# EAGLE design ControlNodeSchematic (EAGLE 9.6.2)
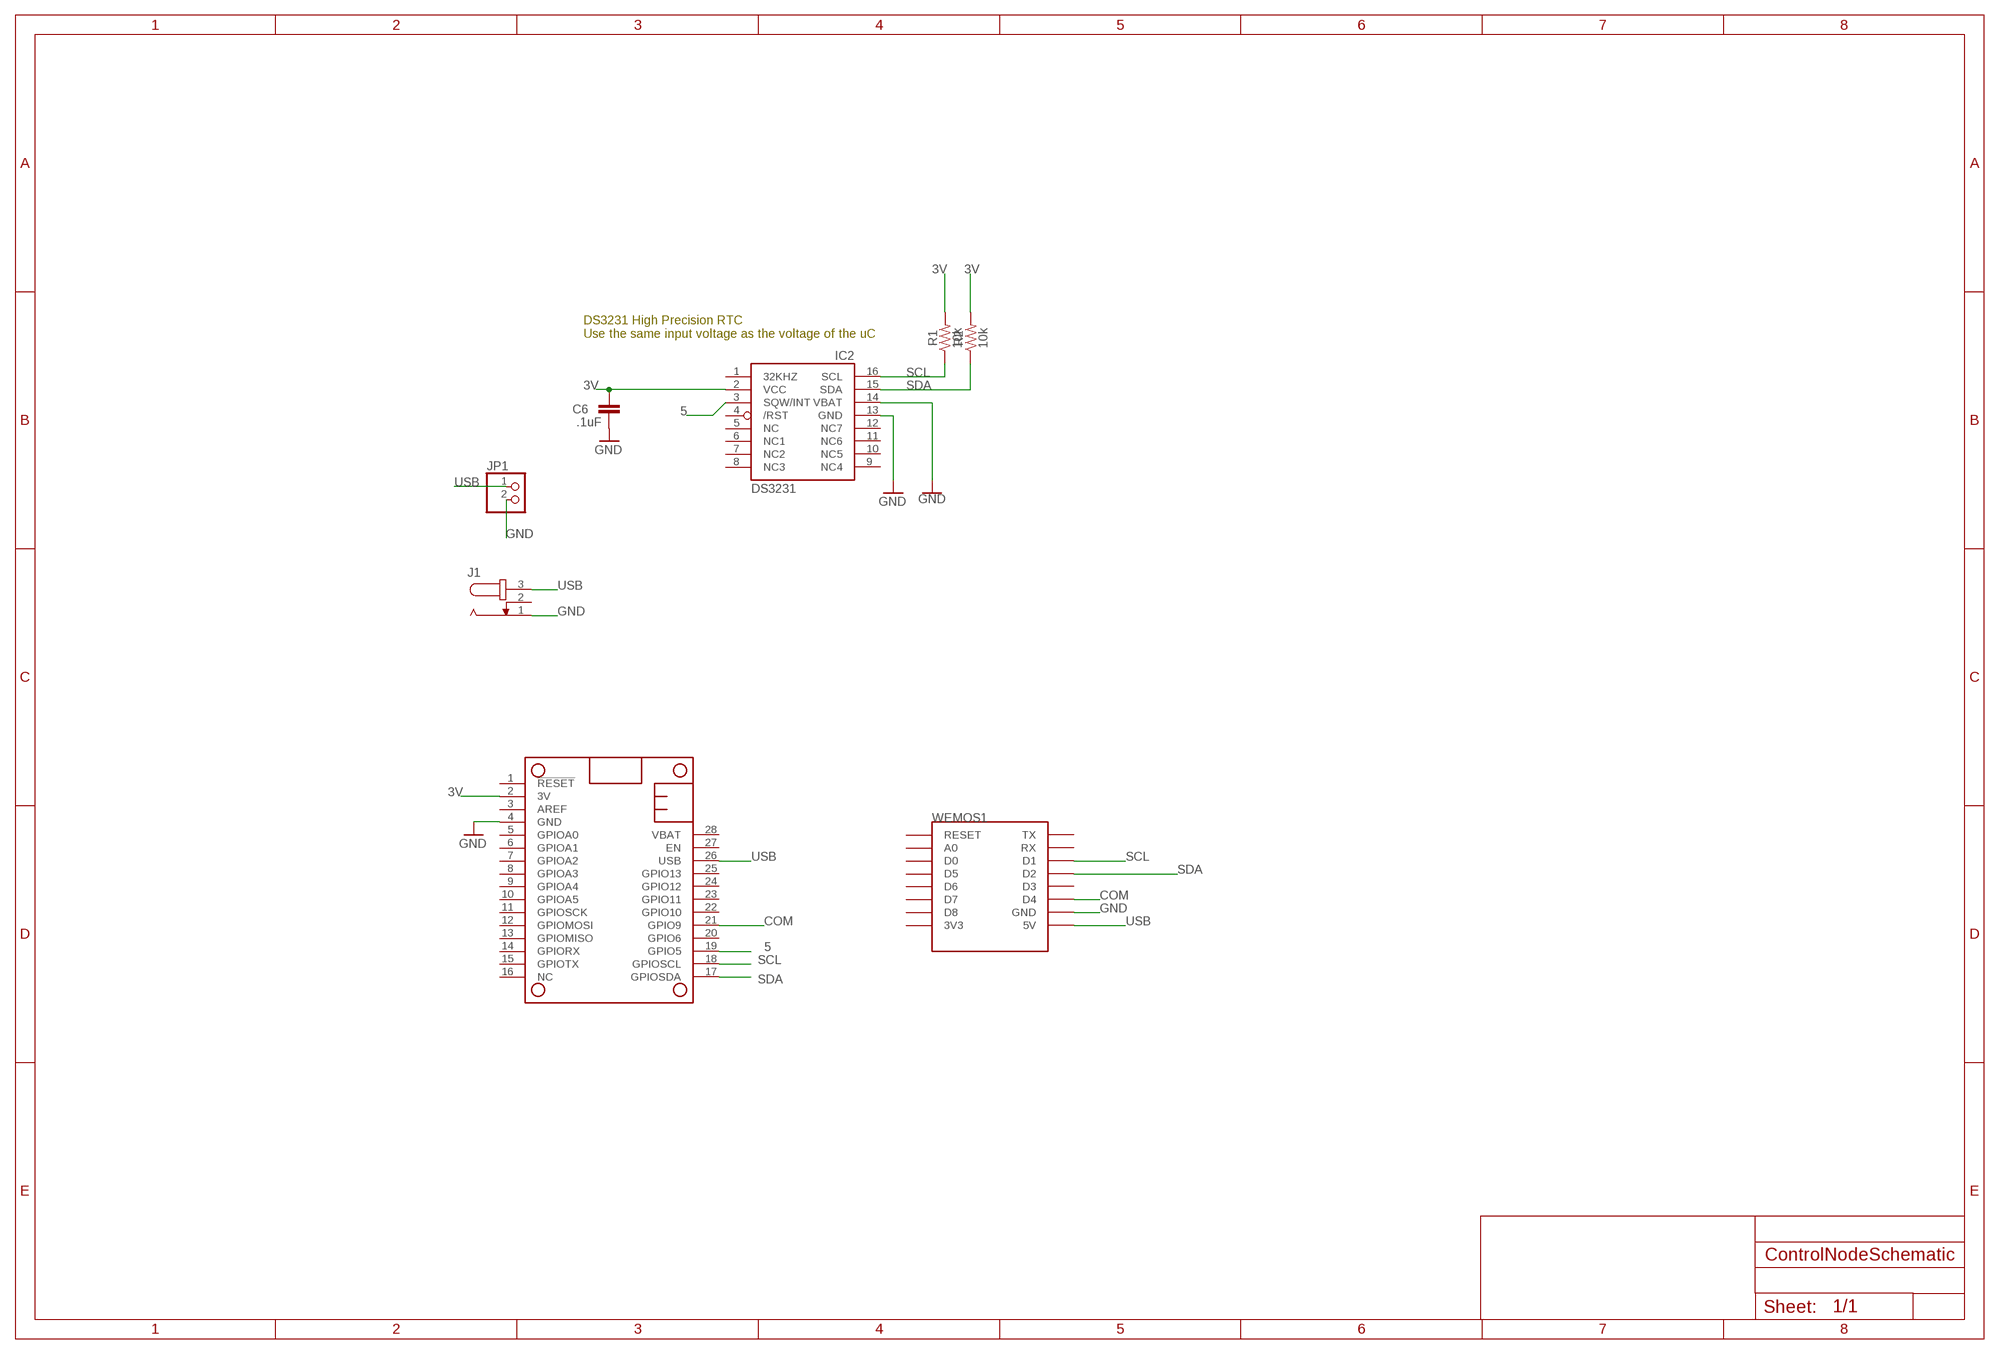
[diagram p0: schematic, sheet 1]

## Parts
C6  .1uF  CC1206  [C1206]
IC2  DS3231/SO  [SO16W]
J1  JACK-PLUG1  [SPC4078]
JP1  PINHD-1X2  [1X02]
MS1  FEATHERWING_NODIM  [FEATHERWING_DIM]
R1  10k  0.27OHM-0603-1/10W-1%  [0603]
R2  10k  0.27OHM-0603-1/10W-1%  [0603]
WEMOS1  WEMOS-D1-MINI  [WEMOS-D1-MINI]

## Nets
3V: C6.1 IC2.2(VCC) MS1.2(3V) R1.2 R2.2
5: IC2.3(SQW/INT) MS1.19(GPIO5)
COM: MS1.21(GPIO9) WEMOS1.D4
GND: C6.2 IC2.13(GND) IC2.14(VBAT) J1.1 JP1.2 MS1.4(GND) WEMOS1.GND
SCL: IC2.16(SCL) MS1.18(GPIOSCL) R1.1 WEMOS1.D1
SDA: IC2.15(SDA) MS1.17(GPIOSDA) R2.1 WEMOS1.D2
USB: J1.3 JP1.1 MS1.26(USB) WEMOS1.5V
Unconnected: IC2.1(32KHZ) IC2.4(/RST) IC2.5(NC) IC2.6(NC1) IC2.7(NC2) IC2.8(NC3) IC2.9(NC4) IC2.10(NC5) IC2.11(NC6) IC2.12(NC7) J1.2 MS1.1(!RESET) MS1.3(AREF) MS1.5(GPIOA0) MS1.6(GPIOA1) MS1.7(GPIOA2) MS1.8(GPIOA3) MS1.9(GPIOA4) MS1.10(GPIOA5) MS1.11(GPIOSCK) MS1.12(GPIOMOSI) MS1.13(GPIOMISO) MS1.14(GPIORX) MS1.15(GPIOTX) MS1.16(NC) MS1.20(GPIO6) MS1.22(GPIO10) MS1.23(GPIO11) MS1.24(GPIO12) MS1.25(GPIO13) MS1.27(EN) MS1.28(VBAT) WEMOS1.3V3 WEMOS1.A0 WEMOS1.D0 WEMOS1.D3 WEMOS1.D5 WEMOS1.D6 WEMOS1.D7 WEMOS1.D8 WEMOS1.RESET WEMOS1.RX WEMOS1.TX

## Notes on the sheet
- DS3231 High Precision RTC
  Use the same input voltage as the voltage of the uC

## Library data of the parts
C6 = eagle-ltspice:C: CAPACITOR, European symbol; SPICEMODEL: NONE; SPICEPREFIX: C
IC2 = adafruit:DS3231
J1 = con-jack:JACK-PLUG: DC POWER JACK Power Jack, DC, Right Angle, Through Hole, Rated 5A at 16VDC, PC Terminals Distributor: Farnell (www.Farnell.de) Drawing: 84N1161.pdf / 84N1162.pdf Manufacturer: SPC Technology (www.spctechnology.com) Type: SPC4077 / SPC 4078; OC_FARNELL: unknown; OC_NEWARK: unknown
JP1 = pinhead:PINHD-1X2: PIN HEADER
MS1 = adafruit:FEATHERWING
R1 R2 = SparkFun-Resistors:0.27OHM: 0.27Ω resistor; PROD_ID: RES-08787; VALUE: 0.27
WEMOS1 = esp8266modules:WEMOS-D1-MINI: WeMos.cc D1 mini ESP8266 module

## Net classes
0 default: width 0.203 mm, drill 0.203 mm, clearance 0.178 mm

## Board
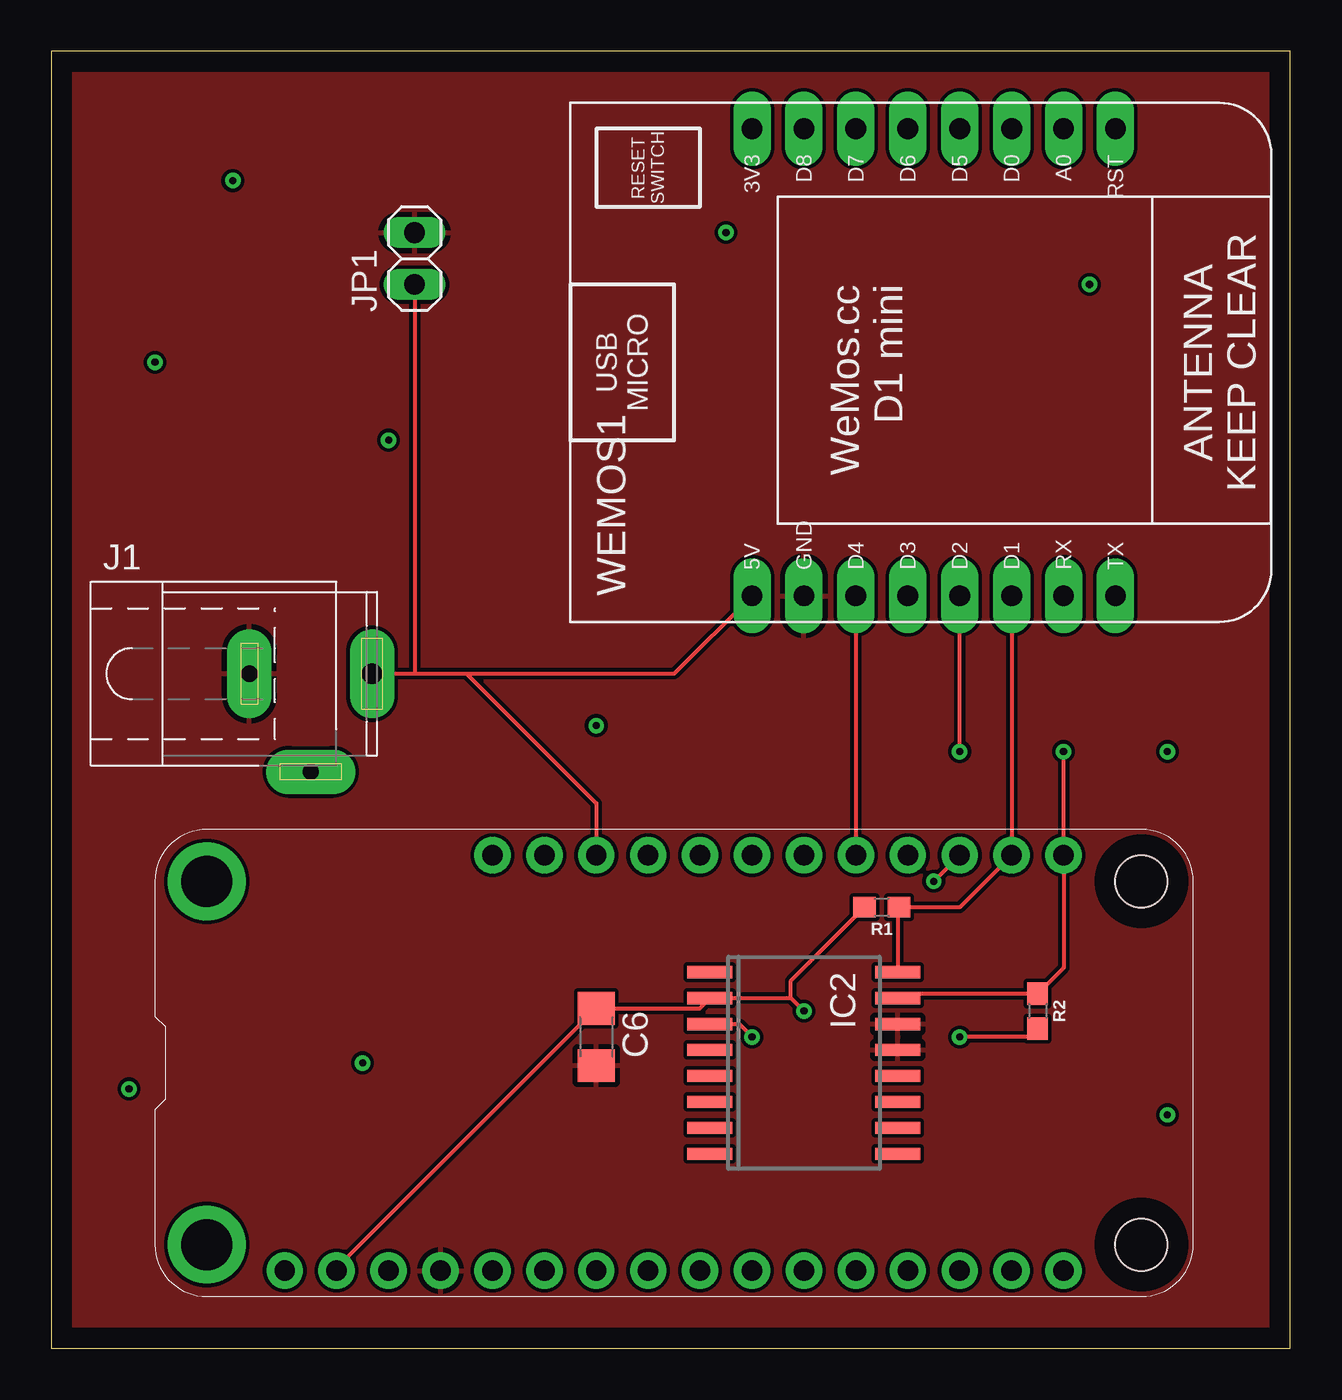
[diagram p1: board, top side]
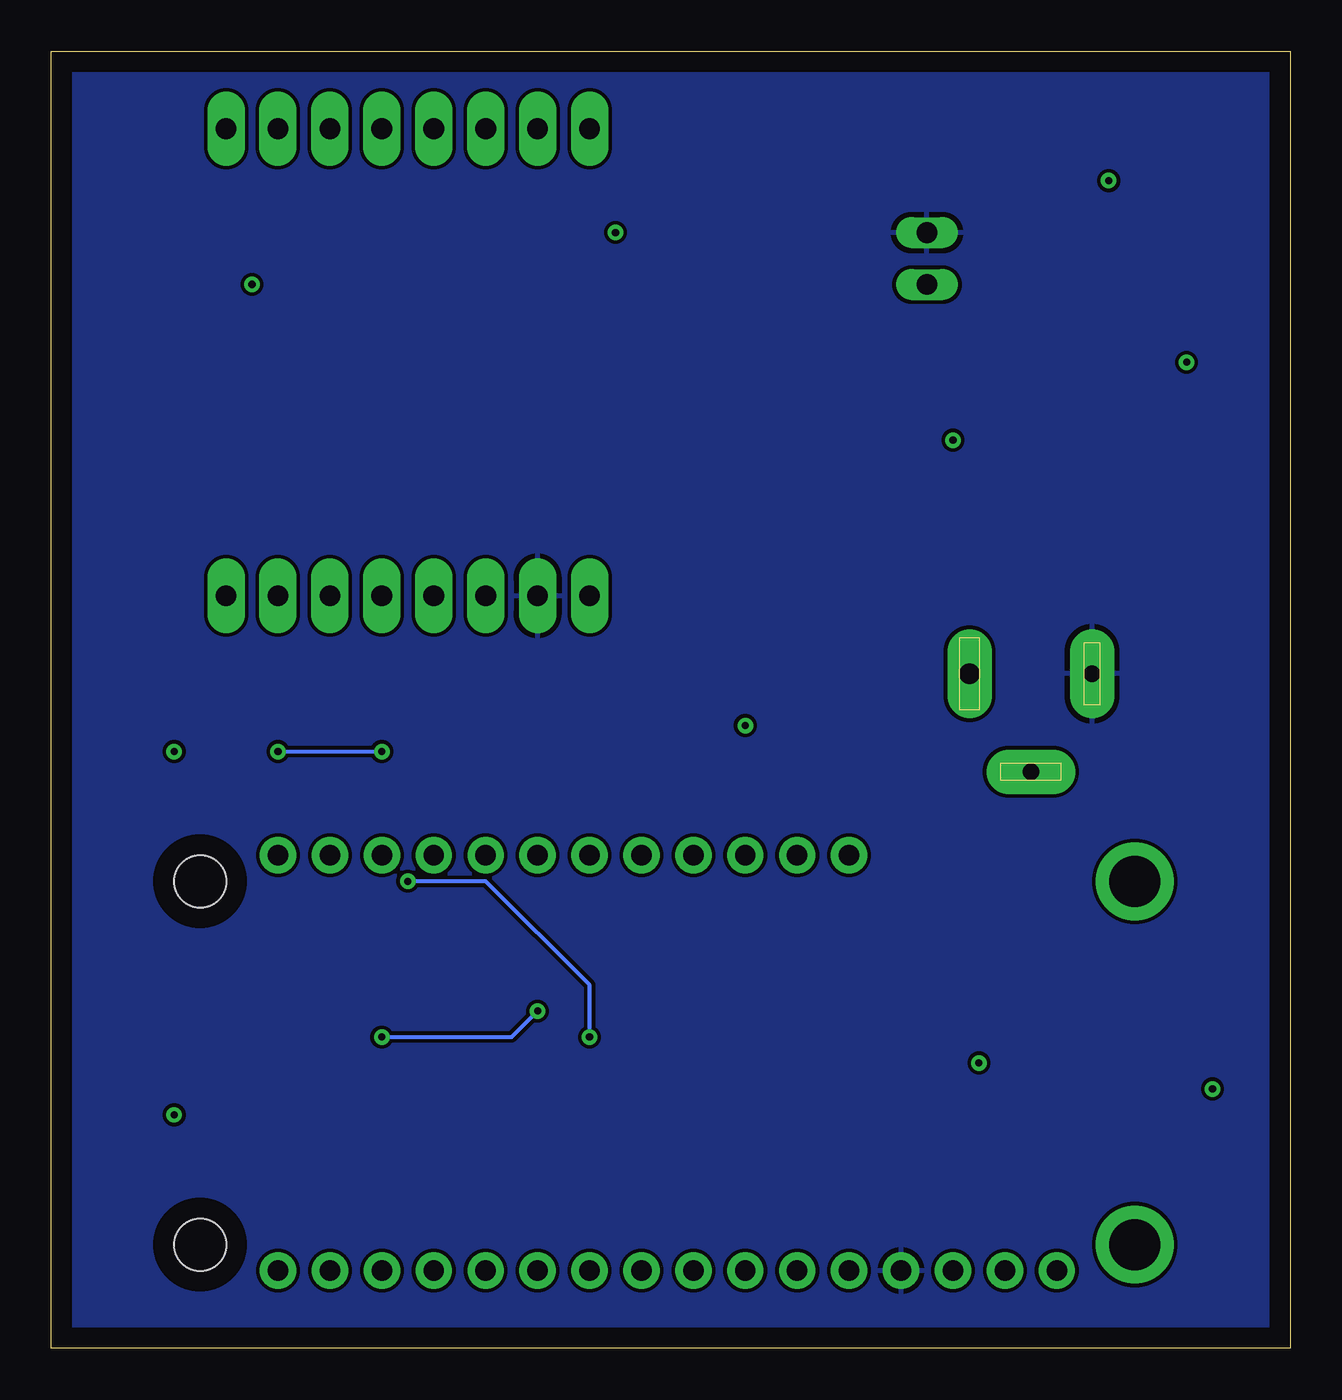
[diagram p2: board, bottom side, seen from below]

Size 60.63 x 63.49 mm. Coordinates in mm from the lower left corner, seen from the top.
Outline: 0,0 60.63,0 60.63,63.49 0,63.49 0,0
Copper layers (1*16): Top 0.035mm / dielectric 1.5mm / Bottom 0.035mm
Design rules "default": minimum track width 6mil, minimum drill 0.35mm, track to track 6mil, track to pad 6mil, pad to pad 6mil, via to via 6mil, smd to smd 6mil, copper to edge 40mil, drill to drill 6mil, minimum pad ring 10mil, minimum via ring 8mil, stop-mask expansion 4mil, vias tented up to drill 0mil, thermal gap 10mil

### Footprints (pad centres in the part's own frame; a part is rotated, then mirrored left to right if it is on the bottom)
C1206 = smd 1.6 x 1.8: 1 -1.4,0; 2 1.4,0
SO16W = smd 0.6 x 2.2: 1 -4.445,-4.6; 2 -3.175,-4.6; 3 -1.905,-4.6; 4 -0.635,-4.6; 5 0.635,-4.6; 6 1.905,-4.6; 7 3.175,-4.6; 8 4.445,-4.6; 9 4.445,4.6; 10 3.175,4.6; 11 1.905,4.6; 12 0.635,4.6; 13 -0.635,4.6; 14 -1.905,4.6; 15 -3.175,4.6; 16 -4.445,4.6
SPC4078 = drill 0.8 pad 2.184 long: 1 -3,0; 2 0,-4.8 | drill 1 pad 2.184 long: 3 3,0
1X02 = drill 1.016 long: 1 -1.27,0; 2 1.27,0
FEATHERWING_DIM = drill 1 pad 1.778: 1 6.35,1.27; 2 8.89,1.27; 3 11.43,1.27; 4 13.97,1.27; 5 16.51,1.27; 6 19.05,1.27; 7 21.59,1.27; 8 24.13,1.27; 9 26.67,1.27; 10 29.21,1.27; 11 31.75,1.27; 12 34.29,1.27; 13 36.83,1.27; 14 39.37,1.27; 15 41.91,1.27; 16 44.45,1.27; 17 44.45,21.59; 18 41.91,21.59; 19 39.37,21.59; 20 36.83,21.59; 21 34.29,21.59; 22 31.75,21.59; 23 29.21,21.59; 24 26.67,21.59; 25 24.13,21.59; 26 21.59,21.59; 27 19.05,21.59; 28 16.51,21.59 | drill 2.5 pad 3.81: P$1 2.54,20.32; P$2 2.54,2.54 | hole 2.54: 48.26,20.32; 48.26,2.54
0603 = smd 1.1 x 1: 1 -0.85,0; 2 0.85,0
WEMOS-D1-MINI = drill 1.016 pad 1.829 long: 3V3 -10.16,-10.16; 5V 12.7,-10.16; A0 -10.16,5.08; D0 -10.16,2.54; D1 12.7,2.54; D2 12.7,0; D3 12.7,-2.54; D4 12.7,-5.08; D5 -10.16,0; D6 -10.16,-2.54; D7 -10.16,-5.08; D8 -10.16,-7.62; GND 12.7,-7.62; RESET -10.16,7.62; RX 12.7,5.08; TX 12.7,7.62

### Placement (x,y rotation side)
C6  26.67,15.24 270 top
IC2  36.83,13.97 270 top
J1  12.7,33.02 0 top
JP1  17.78,53.34 90 top
MS1  5.08,2.54 0 top
R1  40.64,21.59 180 top
R2  48.26,16.51 270 top
WEMOS1  44.45,49.53 270 top

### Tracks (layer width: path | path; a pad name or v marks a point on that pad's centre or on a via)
3V  (via drill 0.35)
  Top 0.203: R2.2 47.84,15.24 v44.45,15.24 | 36.2,17.15 IC2.2 31.73,16.64 C6.1 13.97,3.94 MS1.2 | v36.83,16.51 36.2,17.15 | 36.2,17.15 36.2,17.99 R1.2
  Bottom 0.203: v44.45,15.24 38.1,15.24 v36.83,16.51
5  (via drill 0.35)
  Top 0.203: IC2.3 33.66,15.87 v34.29,15.24 | v43.18,22.86 MS1.19
  Bottom 0.203: v34.29,15.24 34.29,17.78 39.37,22.86 v43.18,22.86
COM
  Top 0.203: WEMOS1.D4 MS1.21
GND
  pour Top: -33.02,74.93 72.39,74.93 72.39,57.15 73.66,55.88 73.66,-7.62 -33.02,-7.62
  pour Bottom: -5.08,69.85 67.31,69.85 67.31,-2.54 -5.08,-2.54
N$1  (via drill 0.35)
  other vias: 8.89,57.15
N$2  (via drill 0.35)
  other vias: 16.51,44.45
N$3  (via drill 0.35)
  other vias: 5.08,48.26
N$4  (via drill 0.35)
  other vias: 15.24,13.97
N$5  (via drill 0.35)
  other vias: 54.61,29.21
N$6  (via drill 0.35)
  other vias: 54.61,11.43
N$7  (via drill 0.35)
  other vias: 50.8,52.07
N$8  (via drill 0.35)
  other vias: 3.81,12.7
N$9  (via drill 0.35)
  other vias: 33.02,54.61
N$10  (via drill 0.35)
  other vias: 26.67,30.48
SCL
  Top 0.203: IC2.16 41.43,21.53 R1.1 44.45,21.59 MS1.18 WEMOS1.D1
SDA  (via drill 0.35)
  Top 0.203: IC2.15 41.65,17.36 R2.1 49.53,18.63 MS1.17 v49.53,29.21 | v44.45,29.21 WEMOS1.D2
  Bottom 0.203: v49.53,29.21 v44.45,29.21
USB
  Top 0.203: J1.3 17.78,33.02 | 17.78,33.02 20.32,33.02 | MS1.26 26.67,26.67 20.32,33.02 | 20.32,33.02 30.48,33.02 WEMOS1.5V | JP1.1 17.78,33.02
